(* Logix 5000 AddOnInstructionDefinition export TeNod4TBlocMain; software revision 28.00 *)

TYPE TeNod4TCAL :   // Calibration datas class 0x65
STRUCT
   MeasureRange : DINT;
   CalibSegments : INT;
   CalibSegment1 : DINT;
   CalibSegment2 : DINT;
   CalibSegment3 : DINT;
   SensorSens : DINT;
   Step : INT;
   CalibZero : DINT;
   CalibCoeff1 : REAL;
   CalibCoeff2 : REAL;
   CalibCoeff3 : REAL;
   CalibSpanCorr : DINT;
   gValueCalib : DINT;
   gValueLocal : DINT;
   ZeroOffset : DINT;
   FixedTare : DINT;
   SensorRef : DINT;
   SensorTol : INT;
END_STRUCT
END_TYPE

TYPE TeNod4TCYCIN :
STRUCT
   eNodCounter : DINT;
   MeasureStatus : TeNod4TStatus;
   Gross : DINT;
   Tare : DINT;
   Net : DINT;
   ADCPoints : DINT;
   CommandEcho : INT;
   Response : INT;
END_STRUCT
END_TYPE

TYPE TeNod4TCYCOUT :
STRUCT
   Command : INT;
END_STRUCT
END_TYPE

TYPE TeNod4TDatas :   // Global datas for eNod4 and functions
STRUCT
   CYCIN : TeNod4TCYCIN;
   CYCOUT : TeNod4TCYCOUT;
   CAL : TeNod4TCAL;
   FIL : TeNod4TFILTER;
   LEGAL : TeNod4TLEGAL;
   IOCFG : TeNod4TIOCFG;
   MSGBuffer : SINT[100];   // Internaly used for explicit messages
   MSGGroup : INT;   // Current message group of last comm error
   MSGClass : INT;   // Current CIP class of last comm error
   MSGAttribute : INT;   // Current CIP attribute of last comm error
   MSGError : INT;   // Last MSG error
   MSGErrorEx : DINT;   // Last MSG extendeed error
   INT : TeNod4TInternal;   // Internal usage
END_STRUCT
END_TYPE

TYPE TeNod4TFILTER :
STRUCT
   ADConversionRate : INT;
   Activation : SINT;
   LowPassOrder : SINT;
   LowPassFreq : INT;
   BandCutHigh : INT;
   BandCutLow : INT;
END_STRUCT
END_TYPE

TYPE TeNod4TInternal :   // For internal usage between blocs, do not use
STRUCT
   CALRead : BOOL;
   CALWrite : BOOL;
   FILTERRead : BOOL;
   FILTERWrite : BOOL;
   CalibWrite : BOOL;
   LegelReadAll : BOOL;
   LegalWriteCfg : BOOL;
   LegalReadLastID : BOOL;
   LegalReadDSD : BOOL;
   LegalWriteID : BOOL;
   IOCFGRead : BOOL;
   IOCFGWrite : BOOL;
   Ready : BOOL;
   Done : BOOL;
   Error : BOOL;
   MSGError : BOOL;
   MSGCancel : BOOL;
   Command : INT;
END_STRUCT
END_TYPE

TYPE TeNod4TIOCFG :
STRUCT
   Input1Function : SINT;
   Input2Function : SINT;
   HoldingTime : INT;
   Output1Function : SINT;
   Output2Function : SINT;
   Output3Function : SINT;
   Output4Function : SINT;
   SetPoint1High : DINT;
   SetPoint1Low : DINT;
   SetPoint2High : DINT;
   SetPoint2Low : DINT;
   SetPoint3High : DINT;
   SetPoint3Low : DINT;
   SetPoint4High : DINT;
   SetPoint4Low : DINT;
   Setpoint12Function : SINT;
   Setpoint34Function : SINT;
END_STRUCT
END_TYPE

TYPE TeNod4TLEGAL :
STRUCT
   eNodVersion : INT;
   ModbusCfg : INT;
   LegalVersion : SINT;
   LegalSwitch : SINT;
   LegalCount : SINT;
   LegalChecksum : INT;
   ZeroConfig : INT;
   Stability : SINT;
   Decimal : SINT;
   Unit : SINT[4];
   DSDLastID : DINT;
   DSDOldestID : DINT;
   DSDCurrentID : DINT;
   DSDReadID : DINT;
   DSDReadNet : DINT;
   DSDResdTare : DINT;
   DSDReadStatus : INT;
   DSDReadChecksum : INT;
   HMIName : SINT[4];
END_STRUCT
END_TYPE

TYPE TeNod4TMSGElement :   // Internal use
STRUCT
   Class : SINT;
   Attribute : SINT;
   Offset : SINT;
   Length : SINT;
END_STRUCT
END_TYPE

TYPE TeNod4TStatus :
STRUCT
   Reserved : INT;
   b00Reserved : BOOL;
   b01Reserved : BOOL;
   b02ErrorCode0 : BOOL;
   b03ErrorCode1 : BOOL;
   b04NoMotion : BOOL;
   b05ZeroWeight : BOOL;
   b06EEPROMFailure : BOOL;
   b07Reserved : BOOL;
   b08Input1ON : BOOL;
   b09Input2ON : BOOL;
   b10Output1ON : BOOL;
   b11Output2ON : BOOL;
   b12Output3ON : BOOL;
   b13Output4ON : BOOL;
   b14TareActive : BOOL;
   b15Reservd : BOOL;
END_STRUCT
END_TYPE

ADD_ON_INSTRUCTION TeNod4TBlocMain   (* revision 1.1, vendor Scaime *)
VAR_IN_OUT
   Datas : TeNod4TDatas; {required}
   DatasIN : SINT[28]; {required}
   DatasOUT : SINT[2]; {required}
   MsgRead : MESSAGE; {required}
   MsgWrite : MESSAGE; {required}
END_VAR
VAR_INPUT
   Zero : BOOL; {visible}
   Tare : BOOL; {visible}
   ResetTare : BOOL; {visible}
   Command : INT; {visible}
END_VAR
VAR_OUTPUT
   Ready : BOOL; {access Read Only, visible}
   Run : BOOL; {access Read Only, visible}
   Done : BOOL; {visible}
   Error : BOOL; {visible}
   Timeout : BOOL; {access Read Only, visible}
END_VAR
VAR_INPUT
   StabWeight : DINT; {visible}
   StabTime : DINT; {visible}
END_VAR
VAR_OUTPUT
   Stability : BOOL; {visible}
END_VAR
VAR
   LoopRRun : BOOL; {access None}
   LoopAttr : INT; {access None}
   LoopDec : INT := 64; {access None}
   LoopLen : INT := 2; {access None}
   LoopMode : INT; {access None}
   MemCommand : INT; {access None}
   LoopIndex : DINT; {access None}
   LoopEdge : BOOL; {access None}
   LoopRStart : BOOL; {access None}
   LoopRStartEdge : BOOL; {access None}
   LoopRSend : BOOL; {access None}
   IntBuffer : SINT[256]; {access None}
   FirstRun : BOOL; {access None}
   MSGTabCal : TeNod4TMSGElement[20]; {access None}
   LoopTab : TeNod4TMSGElement[50]; {access None}
   MSGTabFilter : TeNod4TMSGElement[10]; {access None}
   LoopRDone : BOOL; {access None}
   CommandEX : BOOL; {access None}
   LoopWStart : BOOL; {access None}
   LoopWStartEdge : BOOL; {access None}
   LoopWRun : BOOL; {access None}
   LoopWSend : BOOL; {access None}
   LoopWDone : BOOL; {access None}
   MSGTabCalib : TeNod4TMSGElement[10] := ([0].Class := 101, [0].Attribute := 2, [0].Offset := 4, [0].Length := 2, [1].Class := 101, [1].Attribute := 3, [1].Offset := 8, [1].Length := 4, [2].Class := 101, [2].Attribute := 4, [2].Offset := 12, [2].Length := 4, [3].Class := 101, [3].Attribute := 5, [3].Offset := 16, [3].Length := 4); {access None}
   TimerReset : TIMER := (PRE := 3000); {access None}
   MSGTabLegalRAll : TeNod4TMSGElement[25]; {access None}
   MSGTabLegalWCfg : TeNod4TMSGElement[10] := ([0].Class := 100, [0].Attribute := 7, [0].Offset := 10, [0].Length := 2, [1].Class := 100, [1].Attribute := 8, [1].Offset := 12, [1].Length := 2, [2].Class := 100, [2].Attribute := 9, [2].Offset := 16, [2].Length := 4, [3].Class := 100, [3].Attribute := 21, [3].Offset := 48, [3].Length := 4); {access None}
   MSGTabLegalRID : TeNod4TMSGElement[2] := ([0].Class := 100, [0].Attribute := 13, [0].Length := 4); {access None}
   MSGTabLegalWID : TeNod4TMSGElement[2] := ([0].Class := 100, [0].Attribute := 15, [0].Length := 4); {access None}
   MSGTabLegalDSD : TeNod4TMSGElement[6]; {access None}
   MemCounter : DINT; {access None}
   TimerOut : TIMER := (PRE := 200); {access None}
   MSGTabIO : TeNod4TMSGElement[20]; {access None}
   TimerStab : TIMER; {access None}
   MemNet : DINT; {access None}
   StabOK : BOOL; {access None}
END_VAR

ROUTINE Logic   (* ladder *)
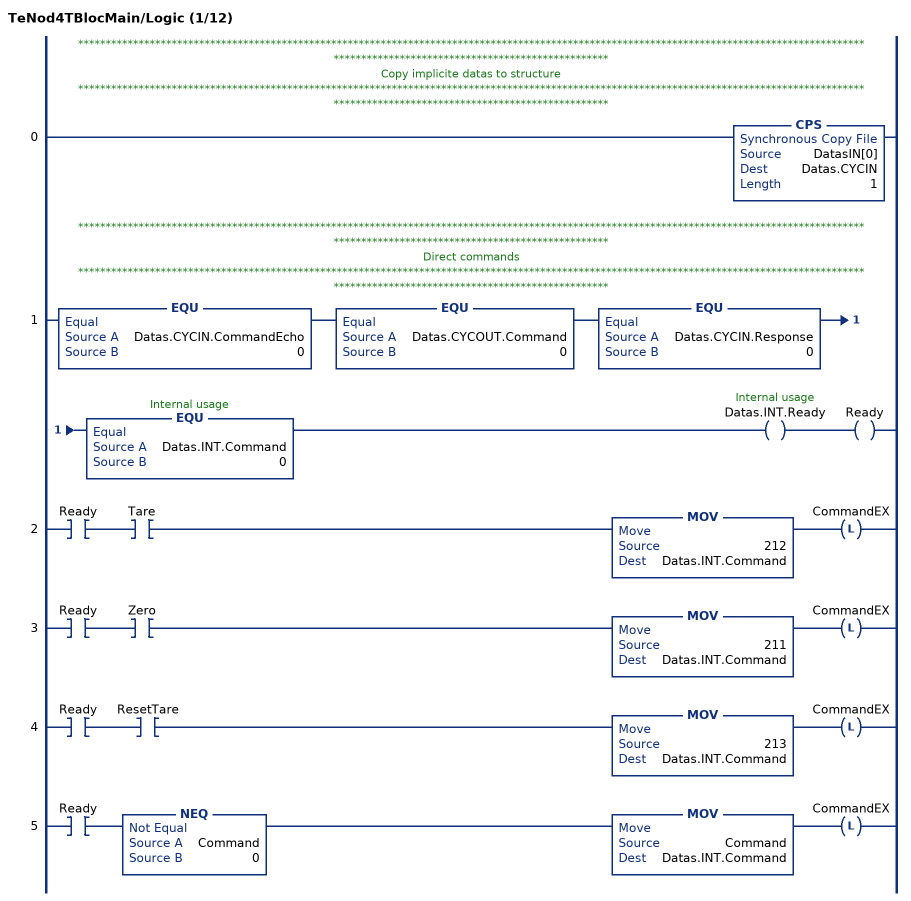
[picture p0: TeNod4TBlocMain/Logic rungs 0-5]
   // *************************************************************************************************************************************************************************************************
   // Copy implicite datas to structure
   // *************************************************************************************************************************************************************************************************
   0: CPS(DatasIN[0],Datas.CYCIN,1);
   // *************************************************************************************************************************************************************************************************
   // Direct commands
   // *************************************************************************************************************************************************************************************************
   1: EQU(Datas.CYCIN.CommandEcho,0)EQU(Datas.CYCOUT.Command,0)EQU(Datas.CYCIN.Response,0)EQU(Datas.INT.Command,0)OTE(Datas.INT.Ready)OTE(Ready);
   2: XIC(Ready)XIC(Tare)MOV(212,Datas.INT.Command)OTL(CommandEX);
   3: XIC(Ready)XIC(Zero)MOV(211,Datas.INT.Command)OTL(CommandEX);
   4: XIC(Ready)XIC(ResetTare)MOV(213,Datas.INT.Command)OTL(CommandEX);
   5: XIC(Ready)NEQ(Command,0)MOV(Command,Datas.INT.Command)OTL(CommandEX);
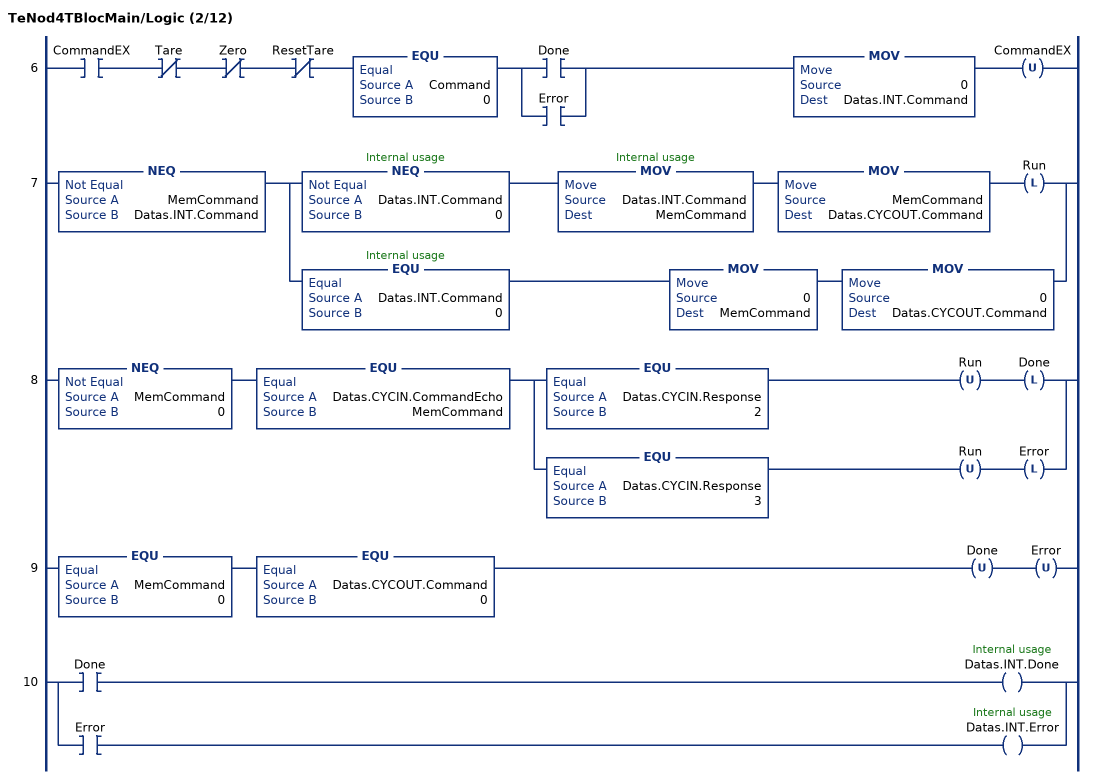
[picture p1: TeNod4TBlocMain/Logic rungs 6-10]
   6: XIC(CommandEX)XIO(Tare)XIO(Zero)XIO(ResetTare)EQU(Command,0)[XIC(Done) ,XIC(Error) ]MOV(0,Datas.INT.Command)OTU(CommandEX);
   7: NEQ(MemCommand,Datas.INT.Command)[NEQ(Datas.INT.Command,0) MOV(Datas.INT.Command,MemCommand) MOV(MemCommand,Datas.CYCOUT.Command) OTL(Run) ,EQU(Datas.INT.Command,0) MOV(0,MemCommand) MOV(0,Datas.CYCOUT.Command) ];
   8: NEQ(MemCommand,0)EQU(Datas.CYCIN.CommandEcho,MemCommand)[EQU(Datas.CYCIN.Response,2) OTU(Run) OTL(Done) ,EQU(Datas.CYCIN.Response,3) OTU(Run) OTL(Error) ];
   9: EQU(MemCommand,0)EQU(Datas.CYCOUT.Command,0)OTU(Done)OTU(Error);
   10: [XIC(Done) OTE(Datas.INT.Done) ,XIC(Error) OTE(Datas.INT.Error) ];
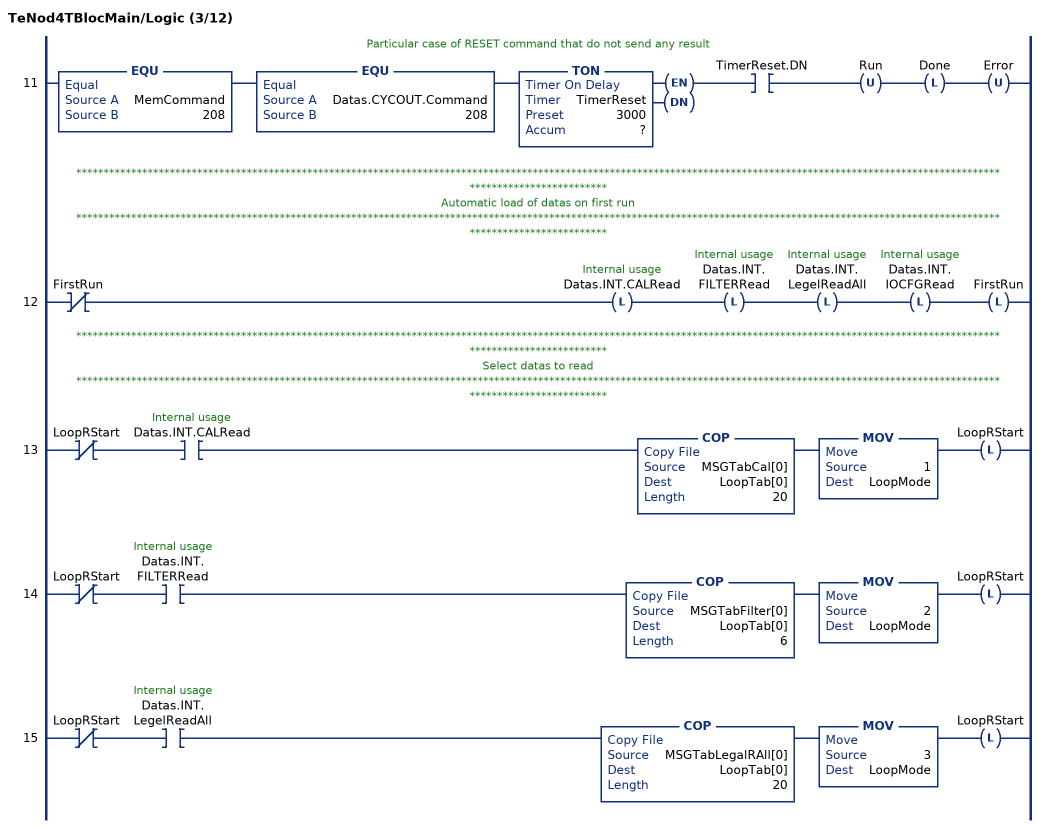
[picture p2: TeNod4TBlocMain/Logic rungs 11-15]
   // Particular case of RESET command that do not send any result
   11: EQU(MemCommand,208)EQU(Datas.CYCOUT.Command,208)TON(TimerReset,?,?)XIC(TimerReset.DN)OTU(Run)OTL(Done)OTU(Error);
   // *************************************************************************************************************************************************************************************************
   // Automatic load of datas on first run
   // *************************************************************************************************************************************************************************************************
   12: XIO(FirstRun)OTL(Datas.INT.CALRead)OTL(Datas.INT.FILTERRead)OTL(Datas.INT.LegelReadAll)OTL(Datas.INT.IOCFGRead)OTL(FirstRun);
   // *************************************************************************************************************************************************************************************************
   // Select datas to read
   // *************************************************************************************************************************************************************************************************
   13: XIO(LoopRStart)XIC(Datas.INT.CALRead)COP(MSGTabCal[0],LoopTab[0],20)MOV(1,LoopMode)OTL(LoopRStart);
   14: XIO(LoopRStart)XIC(Datas.INT.FILTERRead)COP(MSGTabFilter[0],LoopTab[0],6)MOV(2,LoopMode)OTL(LoopRStart);
   15: XIO(LoopRStart)XIC(Datas.INT.LegelReadAll)COP(MSGTabLegalRAll[0],LoopTab[0],20)MOV(3,LoopMode)OTL(LoopRStart);
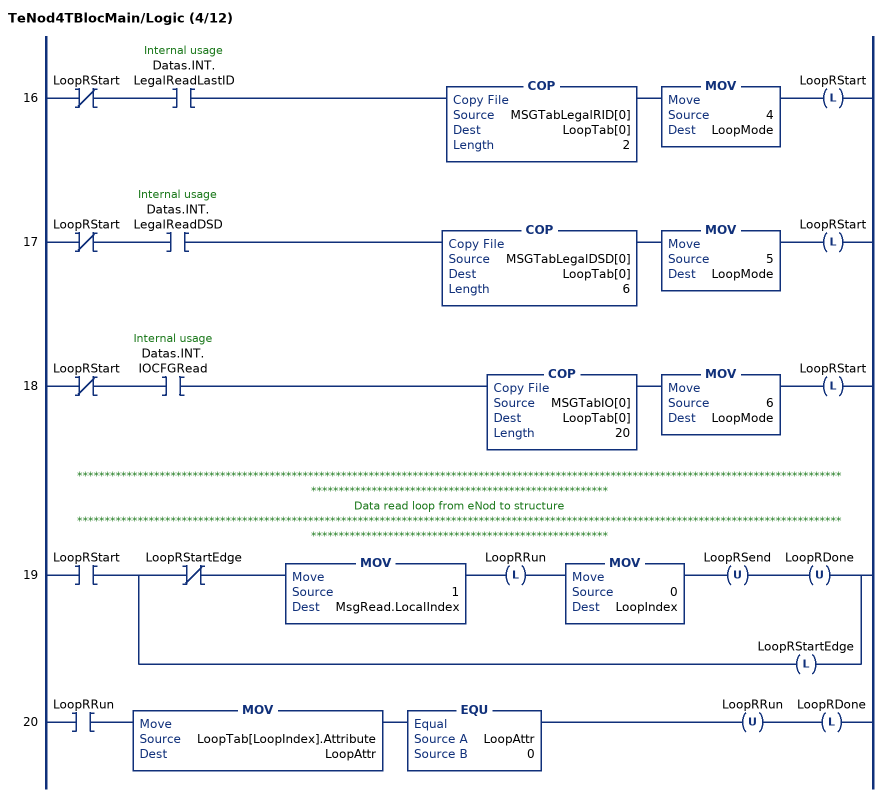
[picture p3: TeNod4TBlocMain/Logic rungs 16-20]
   16: XIO(LoopRStart)XIC(Datas.INT.LegalReadLastID)COP(MSGTabLegalRID[0],LoopTab[0],2)MOV(4,LoopMode)OTL(LoopRStart);
   17: XIO(LoopRStart)XIC(Datas.INT.LegalReadDSD)COP(MSGTabLegalDSD[0],LoopTab[0],6)MOV(5,LoopMode)OTL(LoopRStart);
   18: XIO(LoopRStart)XIC(Datas.INT.IOCFGRead)COP(MSGTabIO[0],LoopTab[0],20)MOV(6,LoopMode)OTL(LoopRStart);
   // *************************************************************************************************************************************************************************************************
   // Data read loop from eNod to structure
   // *************************************************************************************************************************************************************************************************
   19: XIC(LoopRStart)[XIO(LoopRStartEdge) MOV(1,MsgRead.LocalIndex) OTL(LoopRRun) MOV(0,LoopIndex) OTU(LoopRSend) OTU(LoopRDone) ,OTL(LoopRStartEdge) ];
   20: XIC(LoopRRun)MOV(LoopTab[LoopIndex].Attribute,LoopAttr)EQU(LoopAttr,0)OTU(LoopRRun)OTL(LoopRDone);
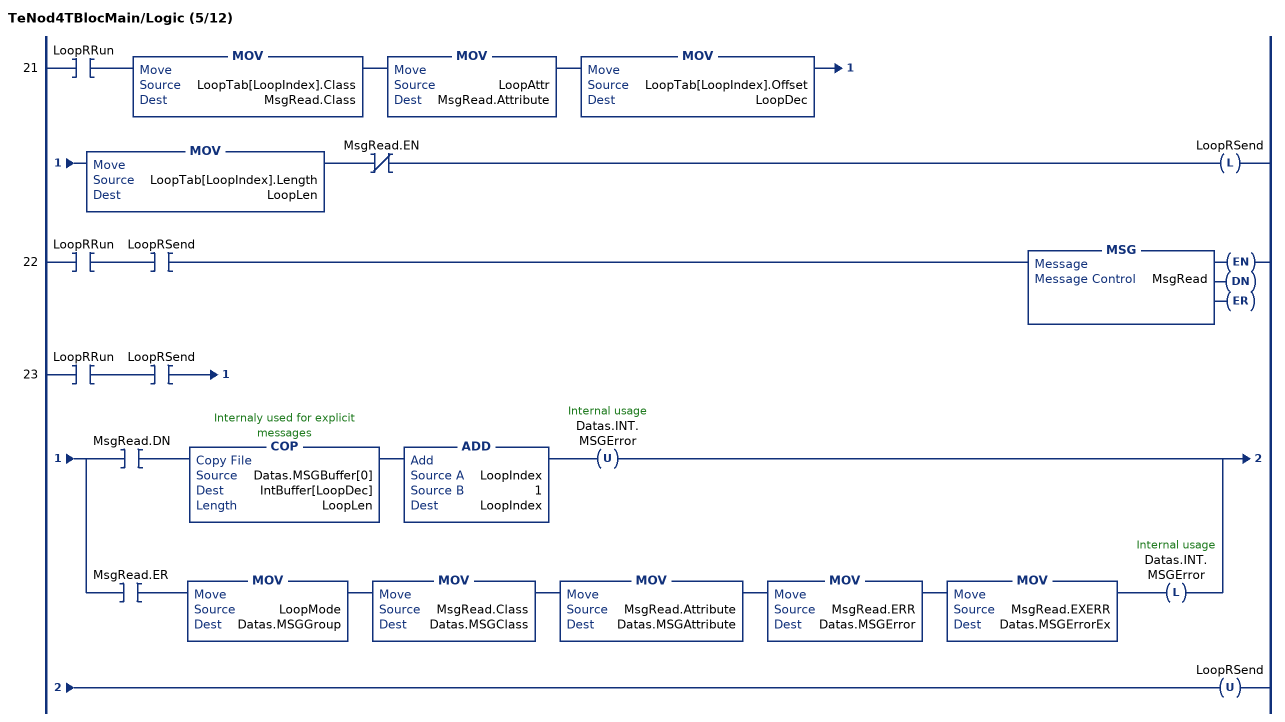
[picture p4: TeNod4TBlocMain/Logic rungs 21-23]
   21: XIC(LoopRRun)MOV(LoopTab[LoopIndex].Class,MsgRead.Class)MOV(LoopAttr,MsgRead.Attribute)MOV(LoopTab[LoopIndex].Offset,LoopDec)MOV(LoopTab[LoopIndex].Length,LoopLen)XIO(MsgRead.EN)OTL(LoopRSend);
   22: XIC(LoopRRun)XIC(LoopRSend)MSG(MsgRead);
   23: XIC(LoopRRun)XIC(LoopRSend)[XIC(MsgRead.DN) COP(Datas.MSGBuffer[0],IntBuffer[LoopDec],LoopLen) ADD(LoopIndex,1,LoopIndex) OTU(Datas.INT.MSGError) ,XIC(MsgRead.ER) MOV(LoopMode,Datas.MSGGroup) MOV(MsgRead.Class,Datas.MSGClass) MOV(MsgRead.Attribute,Datas.MSGAttribute) MOV(MsgRead.ERR,Datas.MSGError) MOV(MsgRead.EXERR,Datas.MSGErrorEx) OTL(Datas.INT.MSGError) ]OTU(LoopRSend);
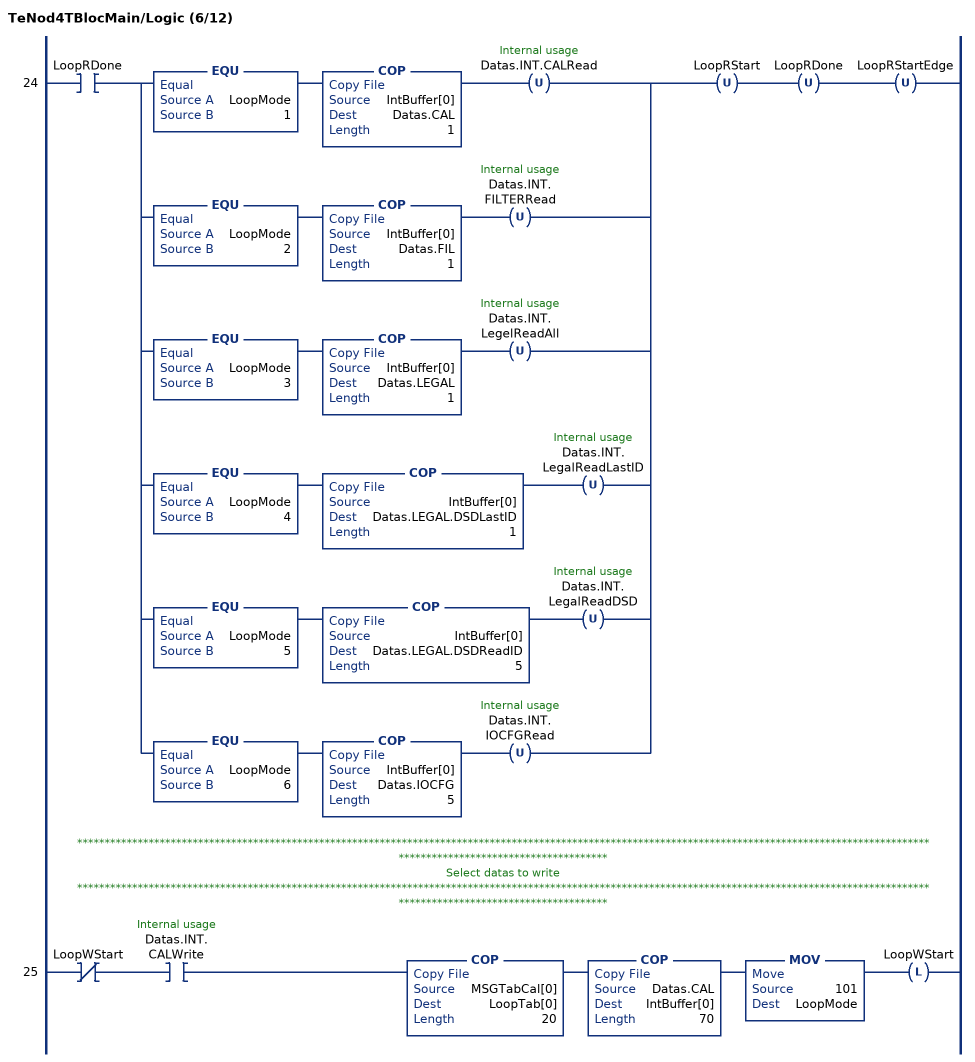
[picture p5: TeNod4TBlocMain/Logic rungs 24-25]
   24: XIC(LoopRDone)[EQU(LoopMode,1) COP(IntBuffer[0],Datas.CAL,1) OTU(Datas.INT.CALRead) ,EQU(LoopMode,2) COP(IntBuffer[0],Datas.FIL,1) OTU(Datas.INT.FILTERRead) ,EQU(LoopMode,3) COP(IntBuffer[0],Datas.LEGAL,1) OTU(Datas.INT.LegelReadAll) ,EQU(LoopMode,4) COP(IntBuffer[0],Datas.LEGAL.DSDLastID,1) OTU(Datas.INT.LegalReadLastID) ,EQU(LoopMode,5) COP(IntBuffer[0],Datas.LEGAL.DSDReadID,5) OTU(Datas.INT.LegalReadDSD) ,EQU(LoopMode,6) COP(IntBuffer[0],Datas.IOCFG,5) OTU(Datas.INT.IOCFGRead) ]OTU(LoopRStart)OTU(LoopRDone)OTU(LoopRStartEdge);
   // *************************************************************************************************************************************************************************************************
   // Select datas to write
   // *************************************************************************************************************************************************************************************************
   25: XIO(LoopWStart)XIC(Datas.INT.CALWrite)COP(MSGTabCal[0],LoopTab[0],20)COP(Datas.CAL,IntBuffer[0],70)MOV(101,LoopMode)OTL(LoopWStart);
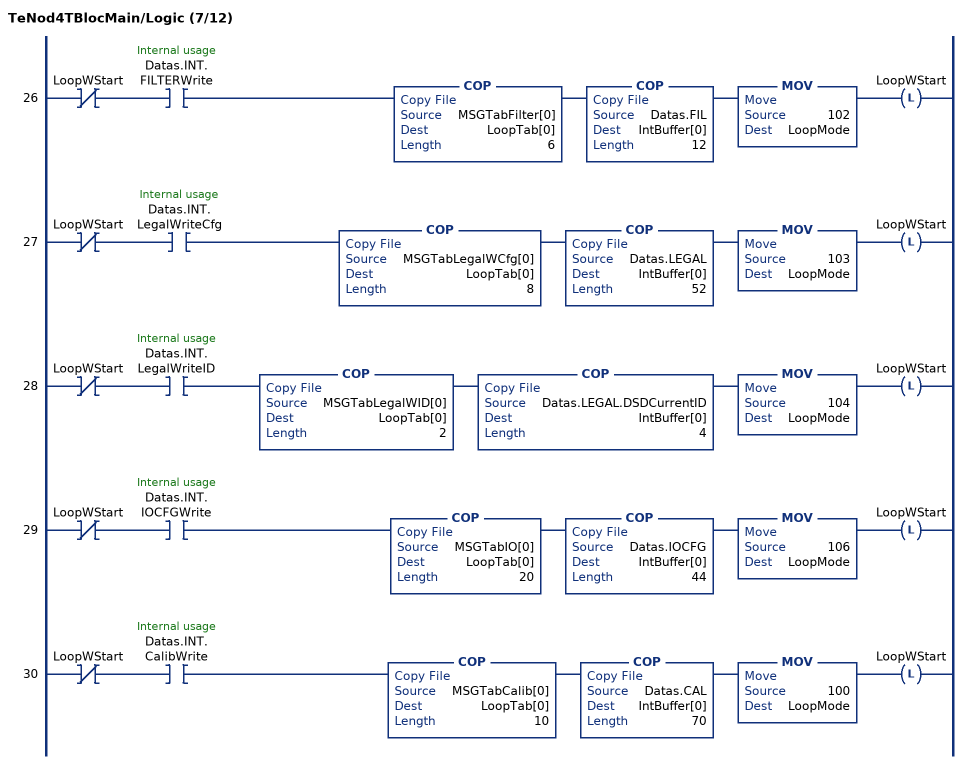
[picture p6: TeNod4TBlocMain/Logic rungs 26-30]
   26: XIO(LoopWStart)XIC(Datas.INT.FILTERWrite)COP(MSGTabFilter[0],LoopTab[0],6)COP(Datas.FIL,IntBuffer[0],12)MOV(102,LoopMode)OTL(LoopWStart);
   27: XIO(LoopWStart)XIC(Datas.INT.LegalWriteCfg)COP(MSGTabLegalWCfg[0],LoopTab[0],8)COP(Datas.LEGAL,IntBuffer[0],52)MOV(103,LoopMode)OTL(LoopWStart);
   28: XIO(LoopWStart)XIC(Datas.INT.LegalWriteID)COP(MSGTabLegalWID[0],LoopTab[0],2)COP(Datas.LEGAL.DSDCurrentID,IntBuffer[0],4)MOV(104,LoopMode)OTL(LoopWStart);
   29: XIO(LoopWStart)XIC(Datas.INT.IOCFGWrite)COP(MSGTabIO[0],LoopTab[0],20)COP(Datas.IOCFG,IntBuffer[0],44)MOV(106,LoopMode)OTL(LoopWStart);
   30: XIO(LoopWStart)XIC(Datas.INT.CalibWrite)COP(MSGTabCalib[0],LoopTab[0],10)COP(Datas.CAL,IntBuffer[0],70)MOV(100,LoopMode)OTL(LoopWStart);
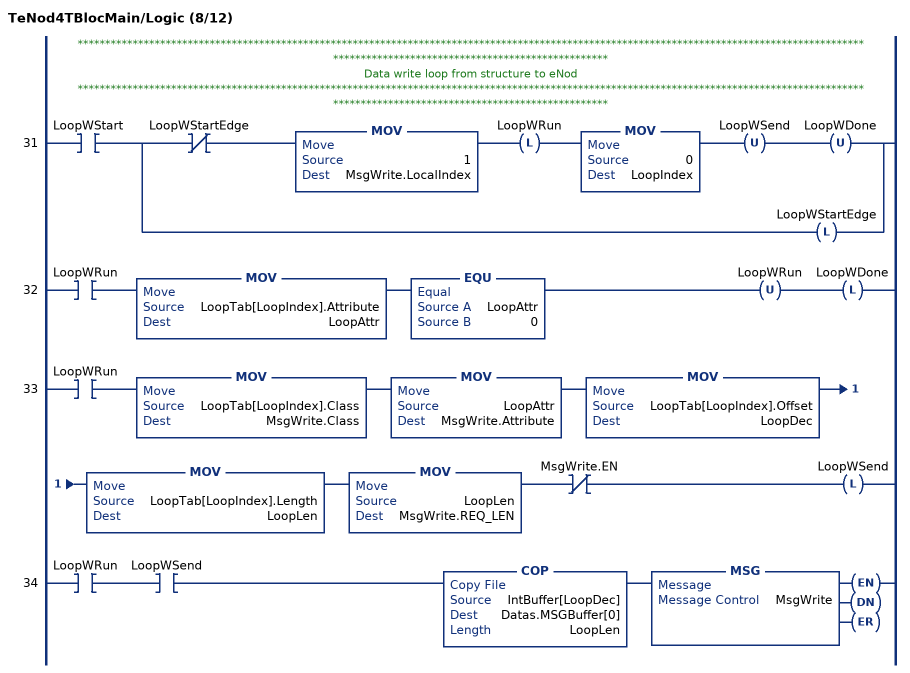
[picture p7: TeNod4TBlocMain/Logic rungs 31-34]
   // *************************************************************************************************************************************************************************************************
   // Data write loop from structure to eNod
   // *************************************************************************************************************************************************************************************************
   31: XIC(LoopWStart)[XIO(LoopWStartEdge) MOV(1,MsgWrite.LocalIndex) OTL(LoopWRun) MOV(0,LoopIndex) OTU(LoopWSend) OTU(LoopWDone) ,OTL(LoopWStartEdge) ];
   32: XIC(LoopWRun)MOV(LoopTab[LoopIndex].Attribute,LoopAttr)EQU(LoopAttr,0)OTU(LoopWRun)OTL(LoopWDone);
   33: XIC(LoopWRun)MOV(LoopTab[LoopIndex].Class,MsgWrite.Class)MOV(LoopAttr,MsgWrite.Attribute)MOV(LoopTab[LoopIndex].Offset,LoopDec)MOV(LoopTab[LoopIndex].Length,LoopLen)MOV(LoopLen,MsgWrite.REQ_LEN)XIO(MsgWrite.EN)OTL(LoopWSend);
   34: XIC(LoopWRun)XIC(LoopWSend)COP(IntBuffer[LoopDec],Datas.MSGBuffer[0],LoopLen)MSG(MsgWrite);
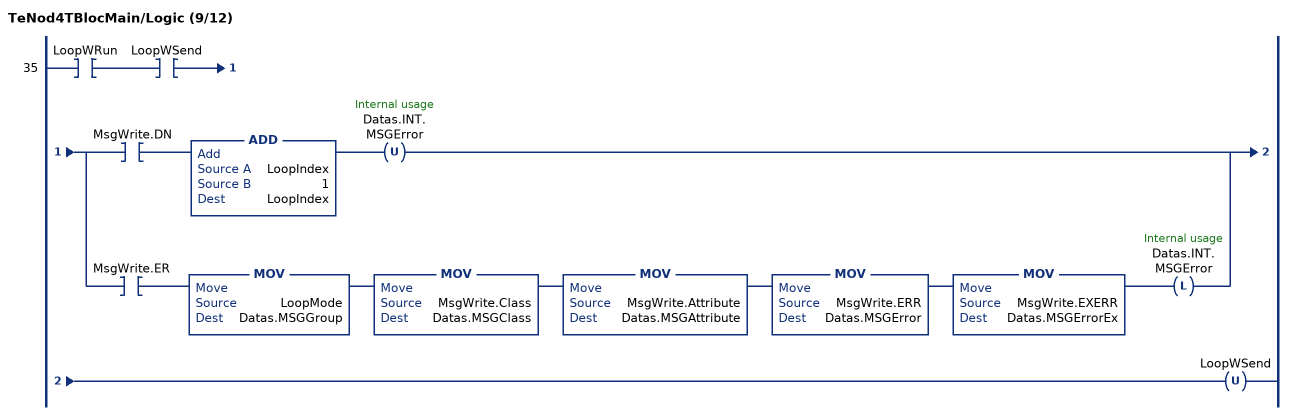
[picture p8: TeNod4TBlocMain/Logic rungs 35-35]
   35: XIC(LoopWRun)XIC(LoopWSend)[XIC(MsgWrite.DN) ADD(LoopIndex,1,LoopIndex) OTU(Datas.INT.MSGError) ,XIC(MsgWrite.ER) MOV(LoopMode,Datas.MSGGroup) MOV(MsgWrite.Class,Datas.MSGClass) MOV(MsgWrite.Attribute,Datas.MSGAttribute) MOV(MsgWrite.ERR,Datas.MSGError) MOV(MsgWrite.EXERR,Datas.MSGErrorEx) OTL(Datas.INT.MSGError) ]OTU(LoopWSend);
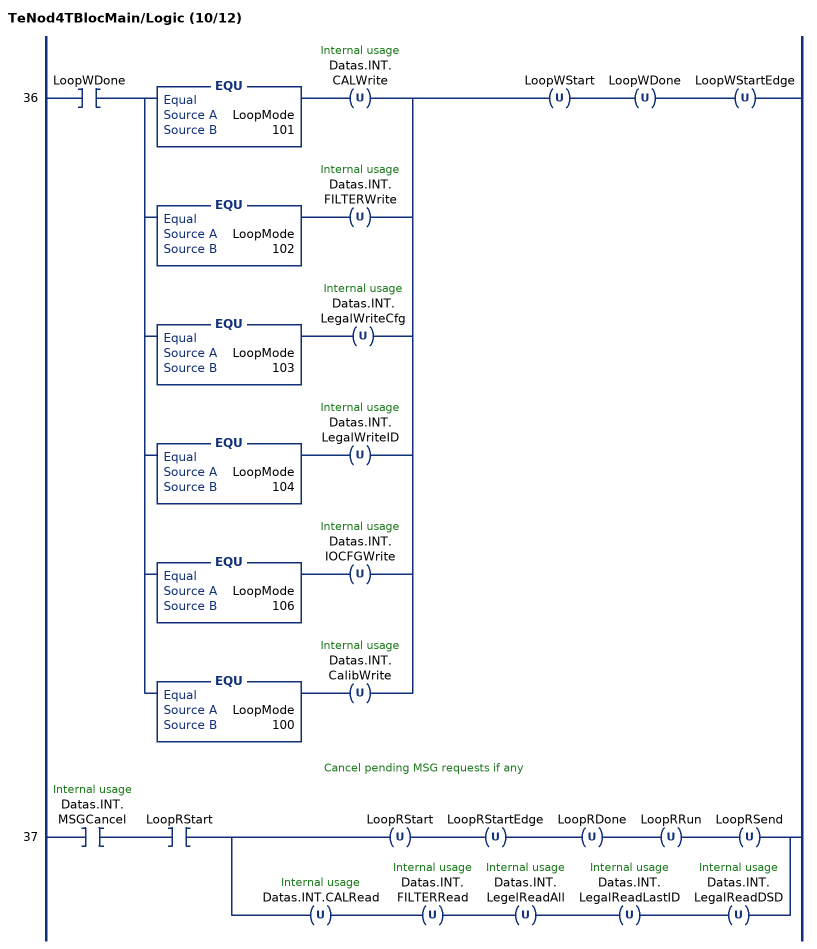
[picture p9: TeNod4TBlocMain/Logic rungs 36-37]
   36: XIC(LoopWDone)[EQU(LoopMode,101) OTU(Datas.INT.CALWrite) ,EQU(LoopMode,102) OTU(Datas.INT.FILTERWrite) ,EQU(LoopMode,103) OTU(Datas.INT.LegalWriteCfg) ,EQU(LoopMode,104) OTU(Datas.INT.LegalWriteID) ,EQU(LoopMode,106) OTU(Datas.INT.IOCFGWrite) ,EQU(LoopMode,100) OTU(Datas.INT.CalibWrite) ]OTU(LoopWStart)OTU(LoopWDone)OTU(LoopWStartEdge);
   // Cancel pending MSG requests if any
   37: XIC(Datas.INT.MSGCancel)XIC(LoopRStart)[OTU(LoopRStart) OTU(LoopRStartEdge) OTU(LoopRDone) OTU(LoopRRun) OTU(LoopRSend) ,OTU(Datas.INT.CALRead) OTU(Datas.INT.FILTERRead) OTU(Datas.INT.LegelReadAll) OTU(Datas.INT.LegalReadLastID) OTU(Datas.INT.LegalReadDSD) ];
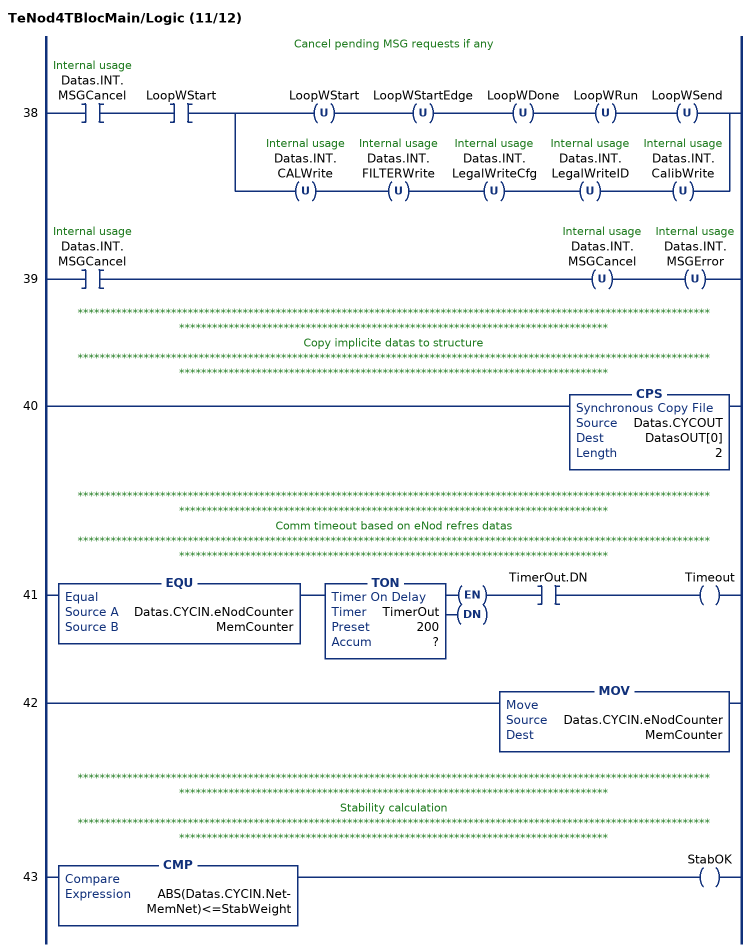
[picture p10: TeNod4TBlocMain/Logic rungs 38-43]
   // Cancel pending MSG requests if any
   38: XIC(Datas.INT.MSGCancel)XIC(LoopWStart)[OTU(LoopWStart) OTU(LoopWStartEdge) OTU(LoopWDone) OTU(LoopWRun) OTU(LoopWSend) ,OTU(Datas.INT.CALWrite) OTU(Datas.INT.FILTERWrite) OTU(Datas.INT.LegalWriteCfg) OTU(Datas.INT.LegalWriteID) OTU(Datas.INT.CalibWrite) ];
   39: XIC(Datas.INT.MSGCancel)OTU(Datas.INT.MSGCancel)OTU(Datas.INT.MSGError);
   // *************************************************************************************************************************************************************************************************
   // Copy implicite datas to structure
   // *************************************************************************************************************************************************************************************************
   40: CPS(Datas.CYCOUT,DatasOUT[0],2);
   // *************************************************************************************************************************************************************************************************
   // Comm timeout based on eNod refres datas
   // *************************************************************************************************************************************************************************************************
   41: EQU(Datas.CYCIN.eNodCounter,MemCounter)TON(TimerOut,?,?)XIC(TimerOut.DN)OTE(Timeout);
   42: MOV(Datas.CYCIN.eNodCounter,MemCounter);
   // *************************************************************************************************************************************************************************************************
   // Stability calculation
   // *************************************************************************************************************************************************************************************************
   43: CMP(ABS(Datas.CYCIN.Net-MemNet)<=StabWeight)OTE(StabOK);
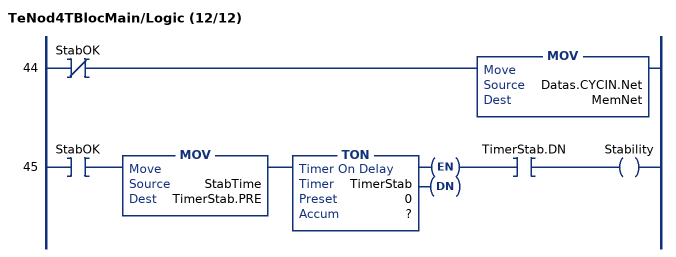
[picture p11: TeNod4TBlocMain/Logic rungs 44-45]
   44: XIO(StabOK)MOV(Datas.CYCIN.Net,MemNet);
   45: XIC(StabOK)MOV(StabTime,TimerStab.PRE)TON(TimerStab,?,?)XIC(TimerStab.DN)OTE(Stability);
END_ROUTINE
END_ADD_ON_INSTRUCTION
